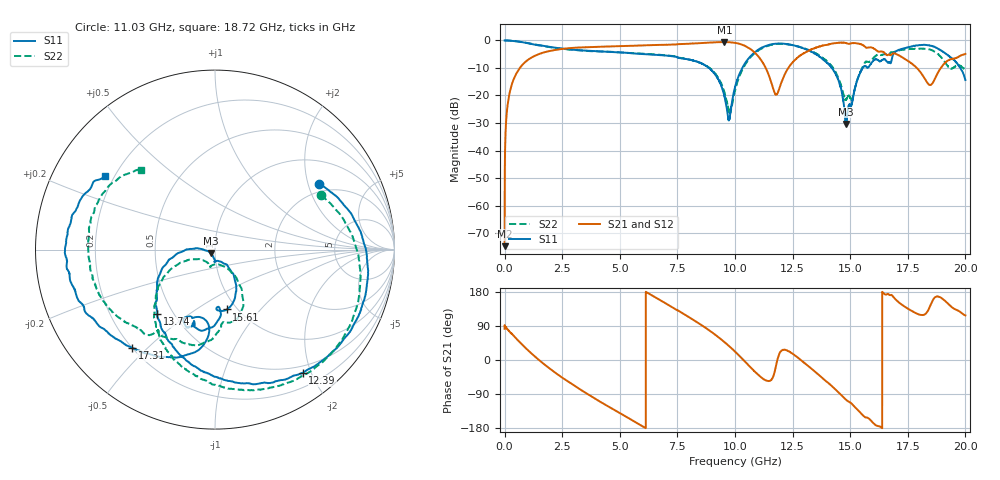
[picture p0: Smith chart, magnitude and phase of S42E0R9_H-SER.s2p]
!{S42E0R9}
!Johanson Technology Inc.
!www.johansontechnology.com
!Test Board Conditions:
!Substrate Type  RO4350B
!Substrate Thickness  50 mil
!Substrate Dk  3.66
!TL Type: GCPW
!TL Trace Width  60 mil
!TL Gap  10 mil
!Electrode orientation  Horizontal
!DUT TOPOLOGY	SERIES
!Mounting Pad LxW  14x55 mil
! Created Wed Nov 25 21:29:28 2020
# khz S ma R 50
! 2 Port Network Data from SP1.SP block
! freq  magS11  angS11  magS21  angS21  magS12  angS12  magS22  angS22
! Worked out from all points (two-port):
!   20001 points, 300 kHz to 20 GHz, reference 50 ohm
!   highest |S21| = -0.57 dB at 9.539 GHz (marker M1); lowest = -74.8 dB at 300 kHz (marker M2)
!   |S21| within 3 dB of the highest: 2.116 GHz to 10.74 GHz (8.622 GHz wide, 134 % of centre); 13.23 GHz to 16.13 GHz (2.902 GHz wide, 19.8 % of centre)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
!   lowest |S11| = -30.3 dB at 14.81 GHz (marker M3), VSWR 1.06, Z = 47.7 - j1.87 ohm
!   |S11| at or under -10 dB: 8.872 GHz to 10.31 GHz (1.443 GHz wide, 15 % of centre); 14.21 GHz to 15.55 GHz (1.341 GHz wide, 9.02 % of centre); 19.78 GHz to end of sweep
!   |S22| runs from -26.4 to 0.0 dB; largest |S21 - S12| = 0.017
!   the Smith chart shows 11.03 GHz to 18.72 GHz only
!   S11 on the Smith chart (normalised r, x): 11.03 GHz: 1.70, +2.36; 12.39 GHz: 0.40, -1.88; 13.74 GHz: 0.41, -0.38; 15.61 GHz: 0.90, -0.68; 17.31 GHz: 0.20, -0.45; 18.72 GHz: 0.16, +0.30
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300  0.9991 -0.2  0.0001828 82.4  4.741e-05 69.0  0.9998 -0.3
128300  0.997 -8.6  0.06596 81.0  0.06625 81.0  0.9975 -8.6
492300  0.9689 -32.6  0.2433 57.5  0.2444 57.6  0.9684 -32.8
1820300  0.78 -105.5  0.6235 -16.1  0.6253 -16.2  0.7734 -106.7
3334300  0.6602 -171.2  0.7469 -79.7  0.7464 -79.8  0.6564 -168.3
6667300  0.545 76.8  0.829 160.9  0.827 160.8  0.5514 66.4
8353300  0.4115 9.0  0.8873 99.6  0.8838 99.7  0.4101 11.2
9539300  0.09863 -31.0  0.936 47.4  0.9369 47.4  0.116 -19.9
9749300  0.03704 32.5  0.9293 36.4  0.9286 36.4  0.04895 19.7
1.00003e7  0.1406 85.9  0.9037 22.3  0.9033 22.3  0.1228 84.9
1.10253e7  0.6864 32.3  0.5053 -40.0  0.503 -39.5  0.6626 27.1
1.17783e7  0.8757 -16.8  0.1036 -16.0  0.104 -15.5  0.8594 -26.9
1.23913e7  0.8428 -54.5  0.3519 20.8  0.3574 20.6  0.837 -65.2
1.33343e7  0.6196 -108.3  0.691 -23.8  0.69 -24.1  0.6312 -113.7
1.37433e7  0.4832 -131.9  0.7931 -44.9  0.7855 -45.1  0.5074 -132.1
1.44313e7  0.2152 -173.7  0.9022 -82.1  0.8987 -81.8  0.234 -157.5
1.48103e7  0.03042 -139.8  0.899 -104.3  0.8969 -104.3  0.08395 -122.5
1.56073e7  0.3397 -79.0  0.7936 -149.4  0.7953 -149.7  0.3751 -67.4
1.66673e7  0.3969 -109.0  0.5548 173.7  0.5446 173.5  0.5563 -125.3
1.73093e7  0.7163 -130.2  0.4803 143.1  0.4726 143.6  0.6808 -154.4
1.87203e7  0.7394 146.3  0.2195 166.9  0.2202 166.8  0.607 132.8
2e7  0.1909 100.1  0.5688 117.8  0.5692 118.5  0.3134 121.2
